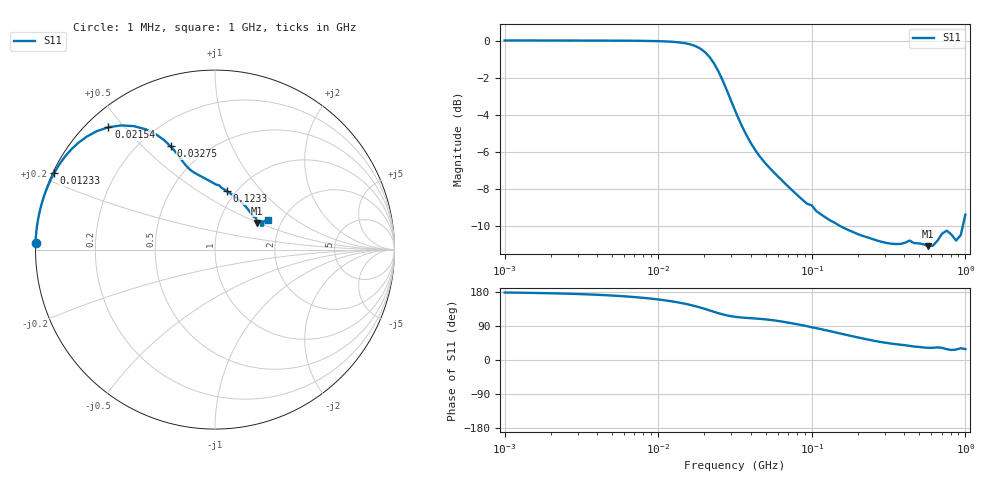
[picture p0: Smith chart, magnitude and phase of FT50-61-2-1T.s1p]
! ListType=Log
!!FT50-61 X 2 1T t2s 12-term
# MHz S RI R 50
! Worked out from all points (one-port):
!   100 points, 1 MHz to 1 GHz, reference 50 ohm
!   lowest |S11| = -11.1 dB at 572.2 MHz (marker M1), VSWR 1.77, Z = 76.1 + j24.5 ohm
!   |S11| at or under -10 dB: 151.6 MHz to 963.4 MHz (811.7 MHz wide, 146 % of centre)
!   S11 on the Smith chart (normalised r, x): 1 MHz: -0.00, +0.02; 12.33 MHz: 0.00, +0.23; 21.54 MHz: 0.06, +0.45; 32.75 MHz: 0.32, +0.61; 123.3 MHz: 0.91, +0.67; 1 GHz: 1.70, +0.63
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1  -1 0.0342
2.477076  -0.9968 0.085
3.764936  -0.9918 0.1293
5.722368  -0.98 0.1967
8.69749  -0.9517 0.2995
12.32847  -0.8968 0.4256
14.17474  -0.8574 0.4891
17.47528  -0.7611 0.5954
18.73817  -0.7141 0.6298
21.54435  -0.5934 0.6818
23.1013  -0.5232 0.6919
24.77076  -0.452 0.6878
28.48036  -0.3282 0.6421
32.74549  -0.2472 0.5754
37.64936  -0.1993 0.5171
46.41589  -0.1526 0.4587
75.64633  -0.0428 0.3895
123.2847  0.0658 0.326
187.3817  0.1425 0.2681
327.4549  0.2055 0.1944
432.8761  0.2295 0.1746
572.2368  0.2357 0.1484
613.5907  0.2366 0.1484
705.4802  0.2555 0.1592
756.4633  0.2694 0.1468
869.749  0.2558 0.1331
932.6033  0.2558 0.1537
1000  0.2969 0.1631
